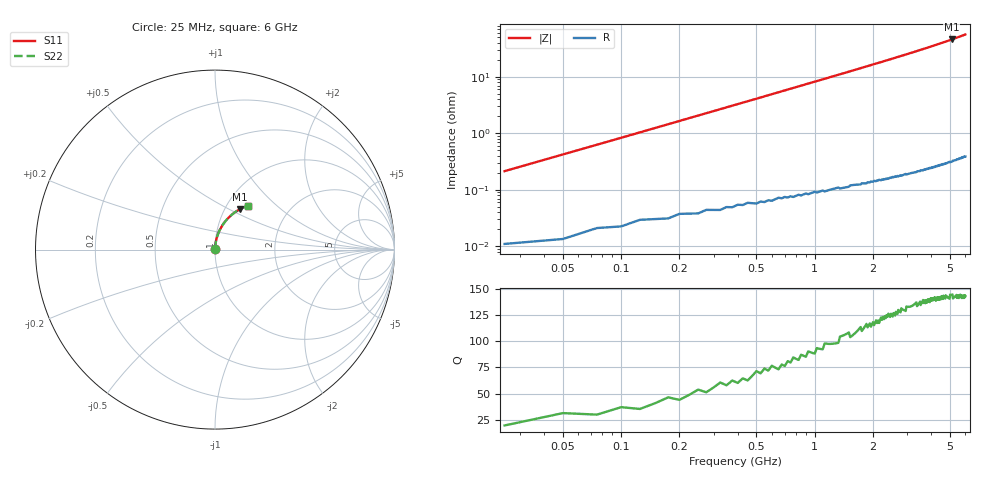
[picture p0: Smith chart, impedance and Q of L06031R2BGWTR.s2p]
!	AVX Thin Film Operation
!	Date:	March	2003
!	Description: Accu-L® Series Thin Film SMD RF Inductors
!	Part Number: L06031R2BGWTR
!	25MHz-6GHz
!	Serial	Measurements
#	mhz	S	db	R	50
!	S11	S11	S21	S21	S12	S12	S22	S22
!	dB	Phase	dB	Phase	dB	Phase	dB	Phase
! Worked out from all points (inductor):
!   240 points, 25 MHz to 6 GHz, reference 50 ohm
!   read as 1/Y11, port 2 shorted: L = 1.34 nH near 50 MHz
!   highest Q = 145 at 5.1 GHz (marker M1), where L = 1.43 nH
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25  -56.59 85.7  -0.00 -0.2  -0.00 -0.2  -56.59 85.7
50  -50.79 86.5  -0.00 -0.3  -0.00 -0.3  -50.79 86.5
75  -47.37 86.8  -0.00 -0.5  -0.00 -0.5  -47.37 86.8
100  -44.93 87.0  -0.00 -0.6  -0.00 -0.6  -44.93 87.0
125  -43.04 87.0  -0.00 -0.8  -0.00 -0.8  -43.04 87.0
175  -40.17 87.0  -0.00 -1.1  -0.00 -1.1  -40.17 87.0
225  -38.03 86.9  -0.00 -1.4  -0.00 -1.4  -38.03 86.9
275  -36.32 86.7  -0.01 -1.7  -0.01 -1.7  -36.32 86.7
325  -34.89 86.5  -0.01 -2.0  -0.01 -2.0  -34.89 86.5
400  -33.11 86.1  -0.01 -2.5  -0.01 -2.5  -33.11 86.1
575  -30.00 85.2  -0.01 -3.6  -0.01 -3.6  -30.00 85.2
775  -27.44 84.1  -0.01 -4.8  -0.01 -4.8  -27.44 84.1
1025  -25.04 82.7  -0.02 -6.4  -0.02 -6.4  -25.04 82.7
1225  -23.51 81.5  -0.03 -7.6  -0.03 -7.6  -23.51 81.5
1475  -21.92 80.0  -0.04 -9.1  -0.04 -9.1  -21.92 80.0
2025  -19.21 76.7  -0.06 -12.5  -0.06 -12.5  -19.21 76.7
2500  -17.42 73.9  -0.09 -15.4  -0.09 -15.4  -17.42 73.9
3025  -15.82 70.7  -0.13 -18.6  -0.13 -18.6  -15.82 70.7
4025  -13.44 64.7  -0.22 -24.7  -0.22 -24.7  -13.44 64.7
5025  -11.64 58.7  -0.33 -30.6  -0.33 -30.6  -11.64 58.7
5100  -11.53 58.2  -0.34 -31.1  -0.34 -31.1  -11.53 58.2
6000  -10.24 52.9  -0.45 -36.4  -0.45 -36.4  -10.24 52.9
